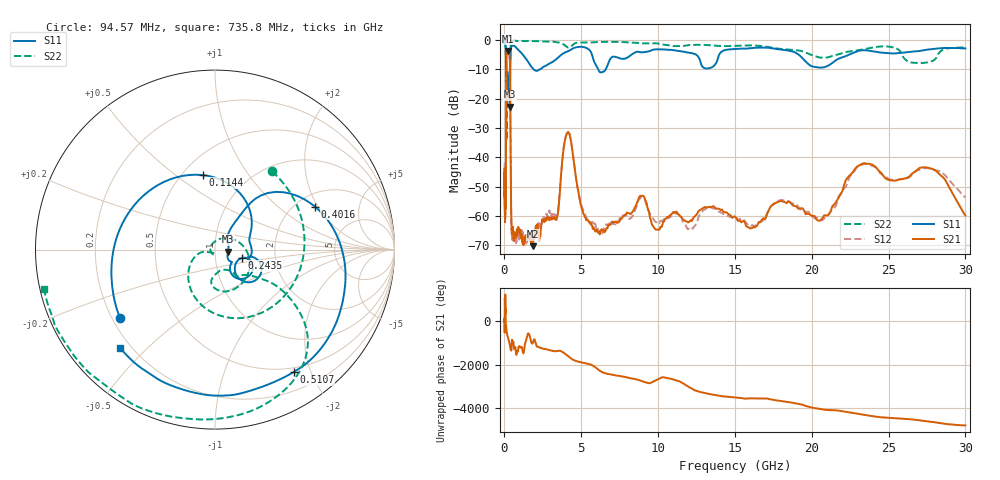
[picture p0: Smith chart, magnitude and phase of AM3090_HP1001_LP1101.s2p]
! Date/Time: Thu, Feb 28, 2019 2:03 PM
! Network Analyzer: Agilent Technologies E8364B Rev: A.07.50.67
! Sweep from 0.010 to 30.000 GHz, 1601 Points, Sweep Type: LOG
! Power Supply: 5.023 V, 0.002 A
# Hz S DB R 50
!freq MagS11 AngS11 MagS21 AngS21 MagS12 AngS12 MagS22 AngS22
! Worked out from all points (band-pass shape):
!   1601 points, 10 MHz to 30 GHz, reference 50 ohm
!   highest |S21| = -3.71 dB at 233.9 MHz (marker M1); lowest = -70.3 dB at 1.839 GHz (marker M2)
!   |S21| within 3 dB of the highest: 125.7 MHz to 347.6 MHz (221.9 MHz wide, 93.8 % of centre)
!   lowest |S11| = -22.7 dB at 340.5 MHz (marker M3), VSWR 1.16, Z = 57.8 - j1.23 ohm
!   |S11| at or under -10 dB: 119.8 MHz to 381.1 MHz (261.4 MHz wide, 104 % of centre); 1.899 GHz to 2.279 GHz (380.3 MHz wide, 18.2 % of centre); 6.102 GHz to 6.588 GHz (486.6 MHz wide, 7.67 % of centre)
!   |S22| runs from -34.3 to -0.1 dB; largest |S21 - S12| = 0.012
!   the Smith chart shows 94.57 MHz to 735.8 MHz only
!   S11 on the Smith chart (normalised r, x): 94.57 MHz: 0.23, -0.31; 114.4 MHz: 0.63, +0.63; 243.5 MHz: 1.35, -0.13; 401.6 MHz: 2.49, +1.89; 510.7 MHz: 0.44, -1.75; 735.8 MHz: 0.16, -0.42
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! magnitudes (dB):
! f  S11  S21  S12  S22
! 10 MHz  -0.3  -45.3  -41.8  -0.7
! 38.04 MHz  -0.5  -60.9  -58.7  -1.6
! 94.57 MHz  -3.7  -44.0  -44.2  -5.4
! 114.4 MHz  -7.5  -14.9  -14.9  -8.5
! 144.7 MHz  -14.0  -4.4  -4.4  -31.8
! 233.9 MHz  -17.1  -3.7  -3.7  -15.3
! 243.5 MHz  -16.0  -3.7  -3.7  -16.0
! 340.5 MHz  -22.7  -6.0  -6.0  -12.5
! 401.6 MHz  -4.3  -36.6  -36.4  -1.1
! 448.4 MHz  -2.3  -61.5  -62.2  -0.4
! 510.7 MHz  -1.8  -64.7  -67.4  -0.2
! 550.5 MHz  -1.8  -63.9  -68.1  -0.2
! 735.8 MHz  -2.4  -66.1  -67.4  -0.2
! 1.839 GHz  -9.6  -70.3  -67.3  -0.3
! 2.084 GHz  -10.5  -63.6  -64.7  -0.4
! 3.385 GHz  -6.4  -61.2  -60.1  -0.7
! 4.115 GHz  -3.8  -31.4  -31.4  -2.5
! 5.338 GHz  -2.7  -61.4  -60.6  -0.8
! 7.926 GHz  -6.2  -59.3  -59.4  -0.7
! 20.41 GHz  -9.3  -61.5  -60.4  -5.8
! 23.59 GHz  -3.5  -42.2  -42.2  -2.9
! 30 GHz  -2.8  -59.8  -53.7  -2.5
